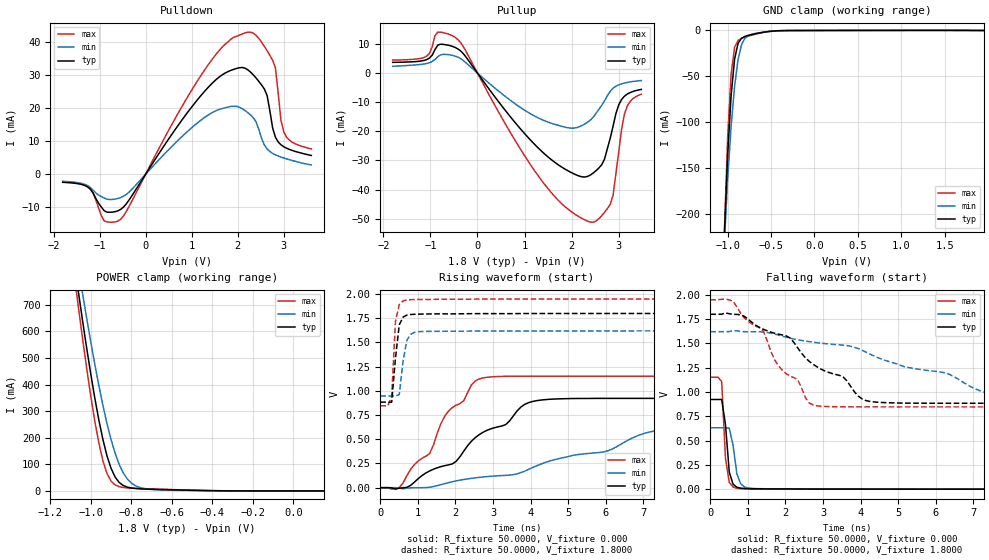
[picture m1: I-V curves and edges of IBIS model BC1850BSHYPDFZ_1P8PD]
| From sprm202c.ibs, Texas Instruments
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|   Model BC1850BSHYPDFZ_1P8PD
[Model]   BC1850BSHYPDFZ_1P8PD
Model_type   I/O
Polarity   Non-Inverting
Enable   Active-Low
Vinl =   0.8500V
Vinh =   0.9800V
Vmeas =   0.9000V
Cref =  15.0000pF
Rref = 100.0000M
Vref =  0.000V
C_comp   1.3000pF   1.4700pF   0.9900pF
[Model Spec]
|   typ   min   max
Vinh   0.98V   0.86V   1.1V
Vinl   0.85V   0.70V   0.91V
[Temperature Range]   25.0000   0.1250k   -40.0000
[Voltage Range]   1.8000V   1.6200V   1.9500V
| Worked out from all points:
|   slope of the pulldown table from 0 to 0.27 V, typ, clamps not added: 46 ohm
|   slope of the pullup table from 0 to 0.27 V, typ, clamps not added: 44.9 ohm
|   GND clamp passes 1 mA (typ) near -0.52 V on its own axis
|   POWER clamp passes 1 mA (typ) near -0.39 V on its own axis
|   rising waveform, R_fixture 50.0000, V_fixture 0.000: 20-80 % time 2.15ns typ, 3.39ns min, 1.36ns max; typ from 0 V to 0.922 V
|   rising waveform, R_fixture 50.0000, V_fixture 1.8000: 20-80 % time 142ps typ, 150ps min, 89.9ps max; typ from 0.883 V to 1.8 V
|   falling waveform, R_fixture 50.0000, V_fixture 0.000: 20-80 % time 128ps typ, 164ps min, 113ps max; typ from 0.922 V to 0 V
|   falling waveform, R_fixture 50.0000, V_fixture 1.8000: 20-80 % time 2.11ns typ, 3.4ns min, 1.39ns max; typ from 1.8 V to 0.883 V
[Pulldown]
| voltage   I(typ)   I(min)   I(max)
-1.8V     -2.432mA   -2.13mA    -2.324mA
-1.2V     -4.535mA   -3.994mA   -4.328mA
-900mV    -11.04mA   -7.186mA   -14.12mA
-540mV    -10.64mA   -7.052mA   -13.61mA
1.32V     25.76mA    17.6mA     32.41mA
2.22V     31.69mA    18.71mA    43.1mA
2.58V     25.85mA    8.892mA    38.8mA
2.76V     14.04mA    6.343mA    34.57mA
2.82V     11.26mA    5.911mA    32.25mA
2.94V     8.959mA    5.237mA    16.42mA
3.06V     7.924mA    4.688mA    11.3mA
3.6V      5.706mA    2.822mA    7.711mA
[Pullup]
| voltage   I(typ)   I(min)   I(max)
-1.8V     3.669mA    2.32mA     4.446mA
-1.08V    4.598mA    3.276mA    5.78mA
-840mV    9.631mA    5.639mA    14.06mA
-420mV    8.322mA    5.5mA      11.54mA
1.32V     -26.18mA   -15.62mA   -35.92mA
1.98V     -34.04mA   -18.91mA   -47.41mA
2.4V      -34.97mA   -16.12mA   -51.17mA
2.64V     -31.45mA   -11.07mA   -48.94mA
2.82V     -22.35mA   -6.26mA    -45.06mA
2.88V     -18.23mA   -5.221mA   -41.92mA
3.12V     -7.968mA   -3.432mA   -14.2mA
3.48V     -5.617mA   -2.562mA   -7.289mA
[GND_clamp]
| voltage   I(typ)   I(min)   I(max)
-1.8V     -5.333A    -4.658A    -5.852A
-1.04V    -227mA     -235.1mA   -226.5mA
-1V       -135.9mA   -161.8mA   -116.4mA
-960mV    -70.64mA   -104.3mA   -47.39mA
-920mV    -31.06mA   -60.7mA    -18.2mA
-880mV    -13.96mA   -31.42mA   -10.74mA
-840mV    -8.411mA   -15.42mA   -8.563mA
-800mV    -6.408mA   -8.312mA   -7.264mA
-760mV    -5.281mA   -5.37mA    -6.127mA
-560mV    -1.528mA   -1.553mA   -1.454mA
-440mV    -390.7uA   -531uA     -281uA
1.95V     0A         0A         0A
[POWER_clamp]
| voltage   I(typ)   I(min)   I(max)
-1.8V     5.299A     4.889A     5.644A
-1.08V    850.3mA    929.8mA    802.1mA
-1.06V    742mA      833.5mA    683.7mA
-1.04V    636.9mA    739.4mA    569mA
-1V       438.9mA    559.8mA    355.9mA
-960mV    265.5mA    395.4mA    179mA
-940mV    192.6mA    321mA      112.6mA
-920mV    131.8mA    253.2mA    65.44mA
-880mV    52.35mA    141.8mA    22.62mA
-820mV    14.23mA    45.21mA    11.42mA
-740mV    7.291mA    9.432mA    8.657mA
150mV     0A         0A         0A
[Ramp]
| variable   typ   min   max
dV/dt_r   0.5530/2.1314n   0.3773/3.4585n   0.6904/1.3440n
dV/dt_f   0.5489/2.0868n   0.4029/3.4626n   0.6605/1.3791n
R_load = 50.0000
[Rising Waveform]
R_fixture = 50.0000
V_fixture = 0.000
V_fixture_min = 0.000
V_fixture_max = 0.000
| time   V(typ)   V(min)   V(max)
0s        2.482uV    1.452uV    3.766uV
505.1ps   -4.637mV   -4.243mV   1.14mV
909.1ps   57.57mV    -770.7uV   238.8mV
1.313ns   172.8mV    4.872mV    352.2mV
1.616ns   217.6mV    31.38mV    664.6mV
1.919ns   245.7mV    61.77mV    828.1mV
2.626ns   546.1mV    106.1mV    1.121V
4.242ns   902.7mV    239.3mV    1.151V
7.374ns   921.7mV    590.1mV    1.151V
10ns      921.7mV    628.8mV    1.151V
[Rising Waveform]
R_fixture = 50.0000
V_fixture = 1.8000
V_fixture_min = 1.6200
V_fixture_max = 1.9500
| time   V(typ)   V(min)   V(max)
0s        882.6mV    945.5mV    845.6mV
202ps     883mV      945.5mV    845.8mV
303ps     881.5mV    946mV      937.8mV
404ps     1.336V     945.4mV    1.717V
505.1ps   1.68V      961mV      1.89V
606.1ps   1.761V     1.308V     1.927V
707.1ps   1.781V     1.521V     1.938V
808.1ps   1.787V     1.583V     1.94V
1.01ns    1.791V     1.609V     1.942V
10ns      1.798V     1.619V     1.946V
[Falling Waveform]
R_fixture = 50.0000
V_fixture = 0.000
V_fixture_min = 0.000
V_fixture_max = 0.000
| time   V(typ)   V(min)   V(max)
0s        921.7mV    630.3mV    1.151V
303ps     922.4mV    630.3mV    1.107V
404ps     664.1mV    630.3mV    316.7mV
505.1ps   175.5mV    626.8mV    70.17mV
606.1ps   50.92mV    449.8mV    21.3mV
707.1ps   19.54mV    158.1mV    8.415mV
808.1ps   10.37mV    55.65mV    4.517mV
909.1ps   7.152mV    23.12mV    3.413mV
1.212ns   3.868mV    5.694mV    1.799mV
10ns      5.67uV     137.9uV    3.766uV
[Falling Waveform]
R_fixture = 50.0000
V_fixture = 1.8000
V_fixture_min = 1.6200
V_fixture_max = 1.9500
| time   V(typ)   V(min)   V(max)
0s        1.798V     1.619V     1.946V
606.1ps   1.797V     1.628V     1.932V
1.414ns   1.643V     1.615V     1.623V
1.818ns   1.593V     1.583V     1.267V
2.323ns   1.454V     1.536V     1.125V
2.727ns   1.286V     1.511V     867.6mV
3.535ns   1.152V     1.48V      846.4mV
4.242ns   902.1mV    1.389V     845.7mV
7.475ns   882.7mV    981.3mV    845.6mV
10ns      882.7mV    947.2mV    845.6mV
